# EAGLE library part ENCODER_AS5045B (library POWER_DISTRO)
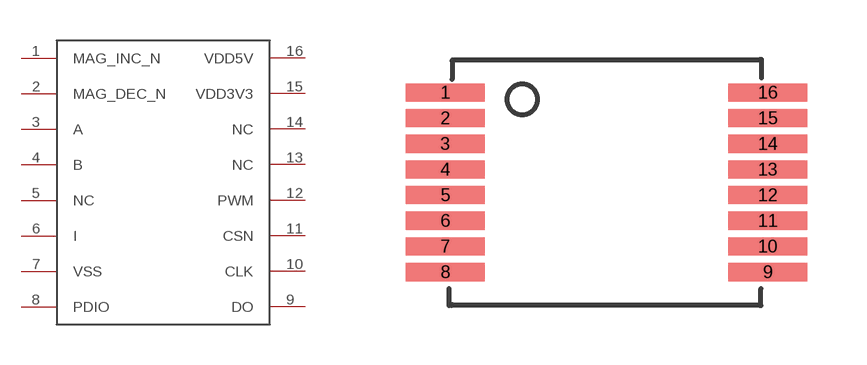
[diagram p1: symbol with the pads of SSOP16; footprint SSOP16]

Designator prefix -

## ENCODER_AS5045B  [SSOP16]
1  MAG_INC_N
2  MAG_DEC_N
3  A
4  B
5  NC
6  I
7  VSS
8  PDIO
9  DO
10  CLK
11  CSN
12  PWM
13  NC
14  NC
15  VDD3V3
16  VDD5V

## Footprint SSOP16 (pad centres in mm)
smd 2 x 0.46: 1 -4.08,2.275; 2 -4.08,1.625; 3 -4.08,0.975; 4 -4.08,0.325; 5 -4.08,-0.325; 6 -4.08,-0.975; 7 -4.08,-1.625; 8 -4.08,-2.275; 9 4.08,-2.275; 10 4.08,-1.625; 11 4.08,-0.975; 12 4.08,-0.325; 13 4.08,0.325; 14 4.08,0.975; 15 4.08,1.625; 16 4.08,2.275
